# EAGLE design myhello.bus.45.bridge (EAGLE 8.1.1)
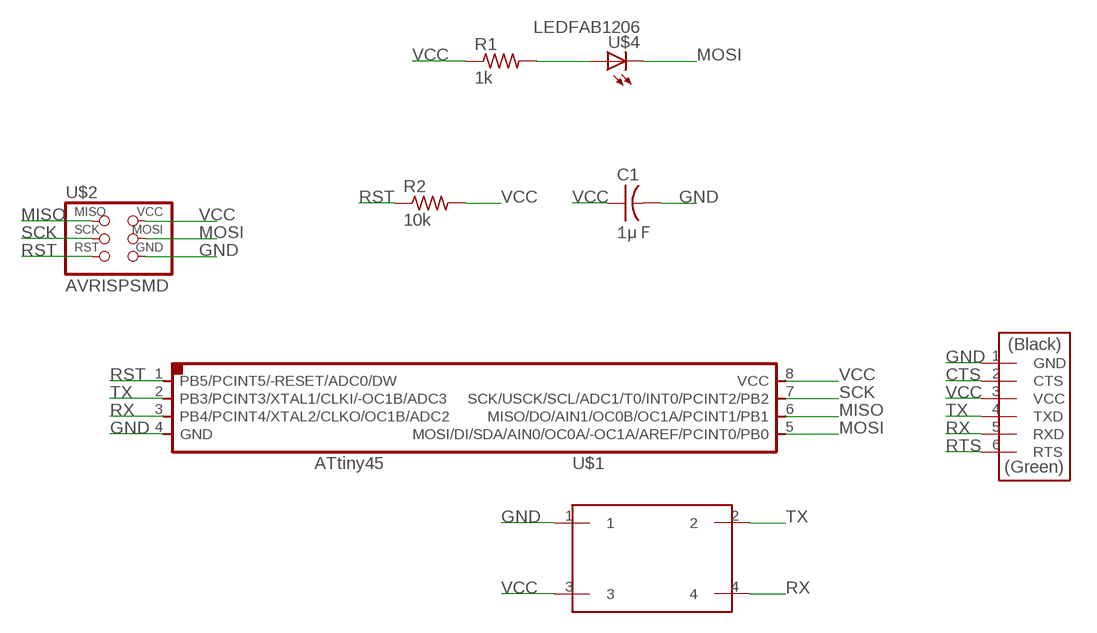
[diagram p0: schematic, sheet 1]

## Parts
C1  1μＦ  CAP-US1206FAB  [C1206FAB]
R1  1k  RES-US1206FAB  [R1206FAB]
R2  10k  RES-US1206FAB  [R1206FAB]
U$1  ATTINY45SI  [SOIC8]
U$2  AVRISPSMD  [2X03SMD]
U$3  FTDI-SMD-HEADER  [1X06SMD]
U$4  LEDFAB1206  [LED1206FAB]
U$5  4PINHEADER2X2  [2X02SMD]

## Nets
CTS: U$3.2(CTS)
GND: C1.2 U$1.4(GND) U$2.6(GND) U$3.1(GND) U$5.1
MISO: U$1.6(MISO/DO/AIN1/OC0B/OC1A/PCINT1/PB1) U$2.1(MISO)
MOSI: U$1.5(MOSI/DI/SDA/AIN0/OC0A/-OC1A/AREF/PCINT0/PB0) U$2.4(MOSI) U$4.2(C)
N$1: R1.2 U$4.1(A)
RST: R2.1 U$1.1(PB5/PCINT5/-RESET/ADC0/DW) U$2.5(RST)
RTS: U$3.6(RTS)
RX: U$1.3(PB4/PCINT4/XTAL2/CLKO/OC1B/ADC2) U$3.5(RXD) U$5.4
SCK: U$1.7(SCK/USCK/SCL/ADC1/T0/INT0/PCINT2/PB2) U$2.3(SCK)
TX: U$1.2(PB3/PCINT3/XTAL1/CLKI/-OC1B/ADC3) U$3.4(TXD) U$5.2
VCC: C1.1 R1.1 R2.2 U$1.8(VCC) U$2.2(VCC) U$3.3(VCC) U$5.3

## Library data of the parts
C1 = fab:CAP-US
R1 R2 = fab:RES-US: Resistor (US Symbol)
U$1 = fab:ATTINY45
U$2 = fab:AVRISP
U$3 = fab:FTDI-SMD-HEADER
U$4 = fab:LED: LED
U$5 = 4pinHeader2X2:4PINHEADER2X2

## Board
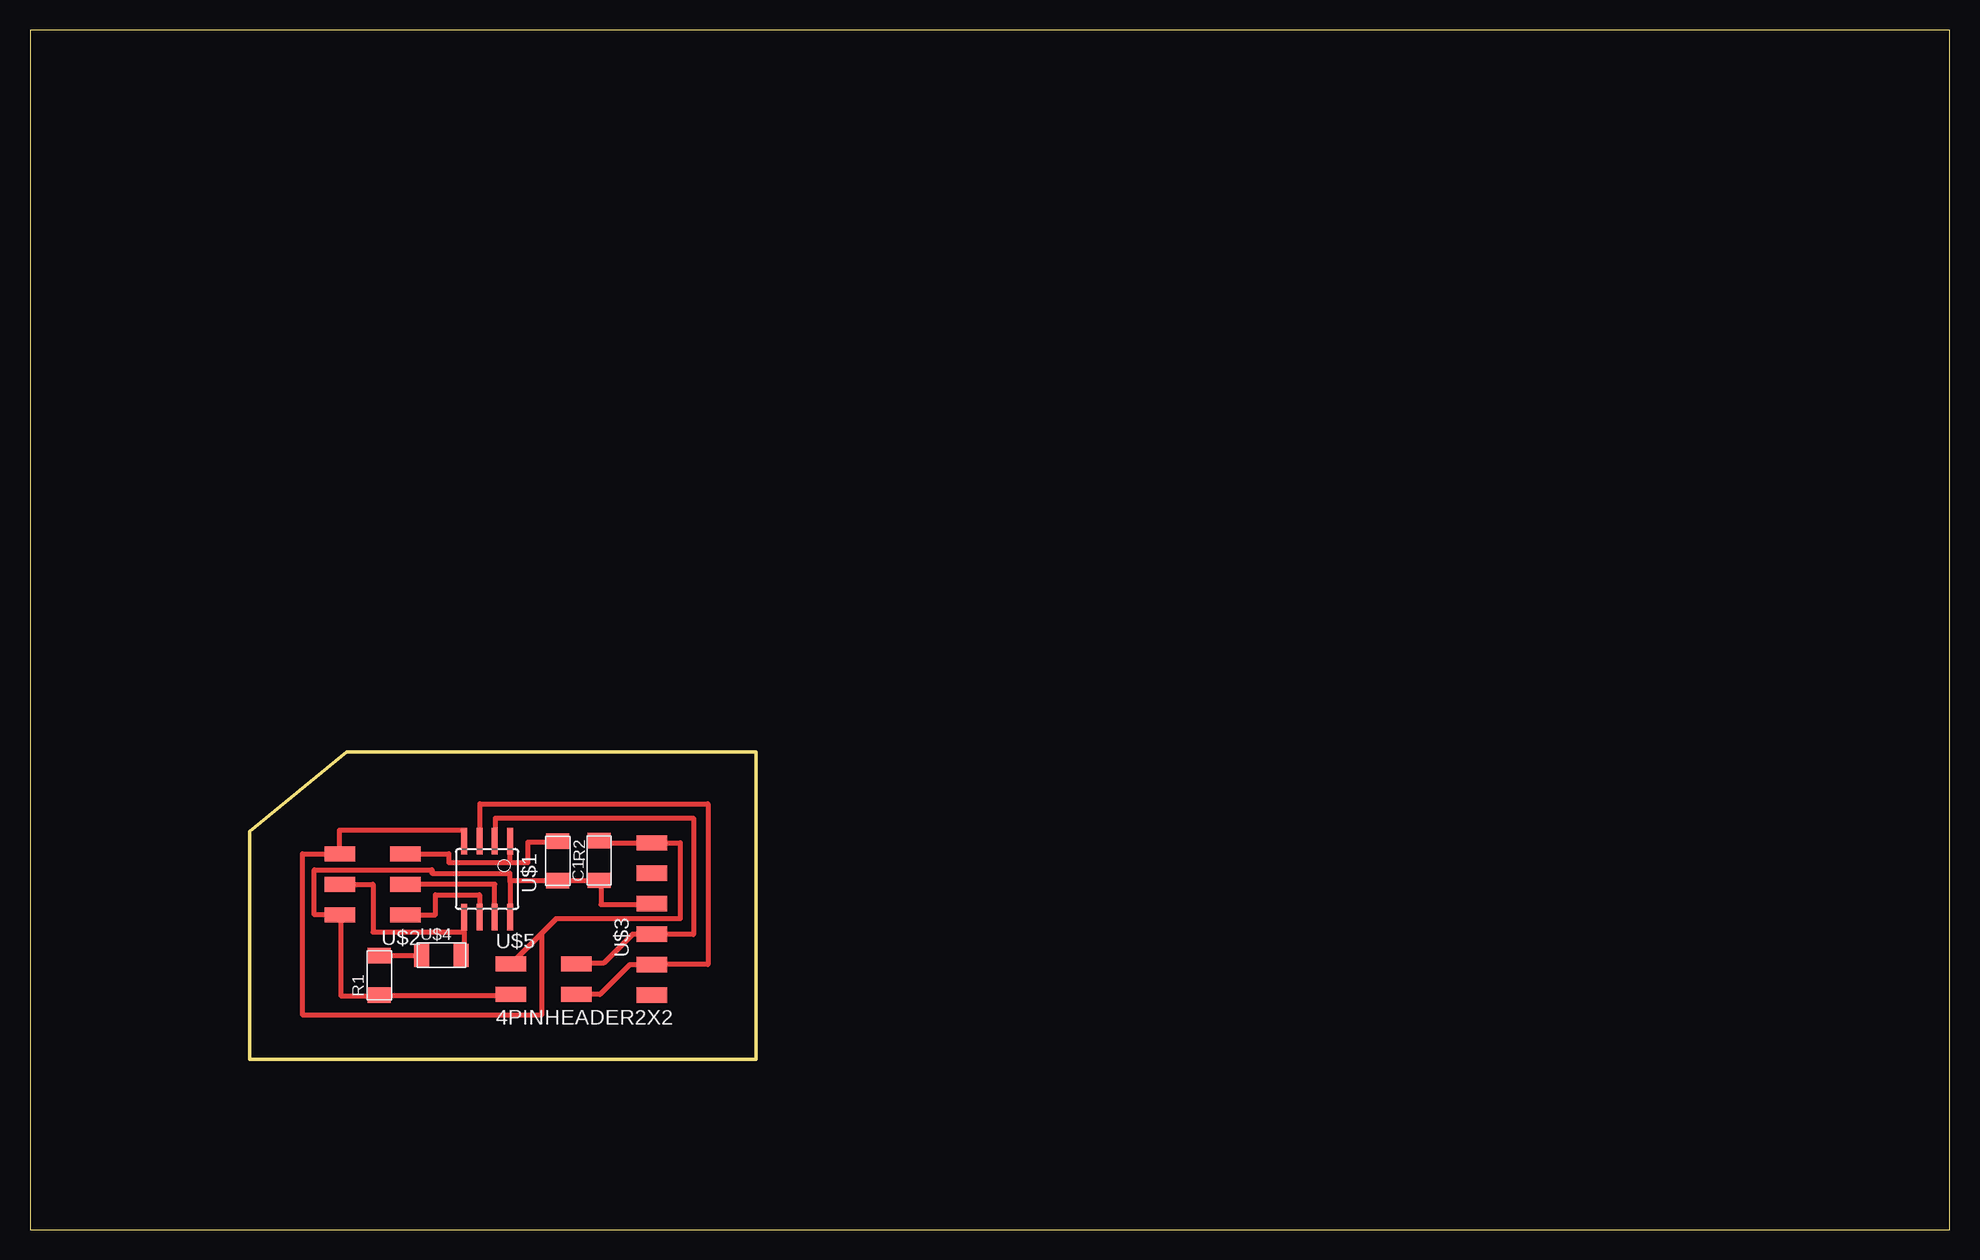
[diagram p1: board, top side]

Size 160 x 100 mm. Coordinates in mm from the lower left corner, seen from the top.
Outline: 0,0 160,0 160,100 0,100 0,0
Outline: 26.4,39.8 60.5,39.8 60.5,14.2 18.3,14.2 18.3,33.2 26.4,39.8
Copper layers (1*16): Top 0.035mm / dielectric 1.5mm / Bottom 0.035mm
Design rules "default": minimum track width 10mil, minimum drill 24mil, track to track 8mil, track to pad 8mil, pad to pad 8mil, via to via 8mil, smd to smd 8mil, copper to edge 40mil, drill to drill 8mil, minimum pad ring 10mil, minimum via ring 8mil, stop-mask expansion 4mil, vias tented up to drill 0mil, thermal gap 10mil

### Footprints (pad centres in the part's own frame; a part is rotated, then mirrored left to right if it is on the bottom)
C1206FAB = smd 1.27 x 1.905: 1 -1.651,0; 2 1.651,0
R1206FAB = smd 1.27 x 1.905: 1 -1.651,0; 2 1.651,0
SOIC8 = smd 0.5 x 2.2: 1 -1.905,-3.154; 2 -0.645,-3.154; 3 0.625,-3.154; 4 1.895,-3.154; 5 1.905,3.154; 6 0.635,3.154; 7 -0.635,3.154; 8 -1.905,3.154
2X03SMD = smd 2.54 x 1.27: 1 -2.54,2.54; 2 2.92,2.54; 3 -2.54,0; 4 2.92,0; 5 -2.54,-2.54; 6 2.92,-2.54
1X06SMD = smd 2.54 x 1.27: 1 0,6.35; 2 0,3.81; 3 0,1.27; 4 0,-1.27; 5 0,-3.81; 6 0,-6.35
LED1206FAB = smd 1.27 x 1.905: 1 -1.651,0; 2 1.651,0
2X02SMD = smd 2.54 x 1.27: 1 -2.54,1.27; 2 2.92,1.27; 3 -2.54,-1.27; 4 2.92,-1.27

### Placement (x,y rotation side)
C1  47.44,30.76 90 top
R1  29.11,21.19 90 top
R2  43.99,30.73 270 top
U$1  38.1,29.21 180 top
U$2  28.77,28.78 180 top
U$3  51.84,25.89 0 top
U$4  34.29,22.86 0 top
U$5  42.63,20.88 0 top

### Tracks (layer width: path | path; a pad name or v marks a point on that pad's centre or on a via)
GND
  Top 0.406: C1.2 47.44,32.24 U$3.1 54.2,32.24 54.2,25.9 43.84,25.9 42.67,24.73 | 42.67,24.73 U$5.1 | 42.67,24.73 42.67,17.9 22.7,17.9 22.7,31.32 U$2.6 25.8,31.32 25.8,33.3 36.2,33.3 U$1.4
MISO
  Top 0.406: U$2.1 33.8,26.24 33.8,27.9 37.47,27.9 U$1.6
MOSI
  Top 0.406: U$4.2 36.2,22.86 36.2,24.7 | 36.2,24.7 U$1.5 | U$2.4 28.6,28.78 28.6,24.8 36.2,24.8 36.2,24.7
N$1
  Top 0.406: R1.2 32.64,22.84 U$4.1
RST
  Top 0.406: U$2.5 34.9,31.32 34.9,30.6 40,30.6 | 40,30.6 41.5,30.6 41.5,32.3 43.99,32.3 R2.1 | 40,30.6 40.01,30.6 U$1.1
RX
  Top 0.406: U$5.4 47.5,19.6 49.98,22.08 U$3.5 51.84,22.1 56.5,22.1 56.5,35.5 37.5,35.5 37.5,32.36 U$1.3
SCK
  Top 0.406: U$1.7 38.73,28.78 U$2.3
TX
  Top 0.406: U$5.2 45.6,22.2 47.8,22.2 50.22,24.62 U$3.4 51.84,24.6 55.3,24.6 55.3,34.3 38.8,34.3 38.8,32.36 U$1.2
VCC
  Top 0.406: U$3.3 51.84,27.1 47.6,27.1 47.6,29.11 C1.1 47.44,29.08 R2.2 40.01,29.08 40.01,29 | U$5.3 40.02,19.54 R1.1 29.11,19.5 25.9,19.5 25.9,26.24 U$2.2 23.7,26.24 23.7,30 33.5,30 33.5,29.7 40.01,29.7 40.01,29 | 40.01,29 U$1.8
